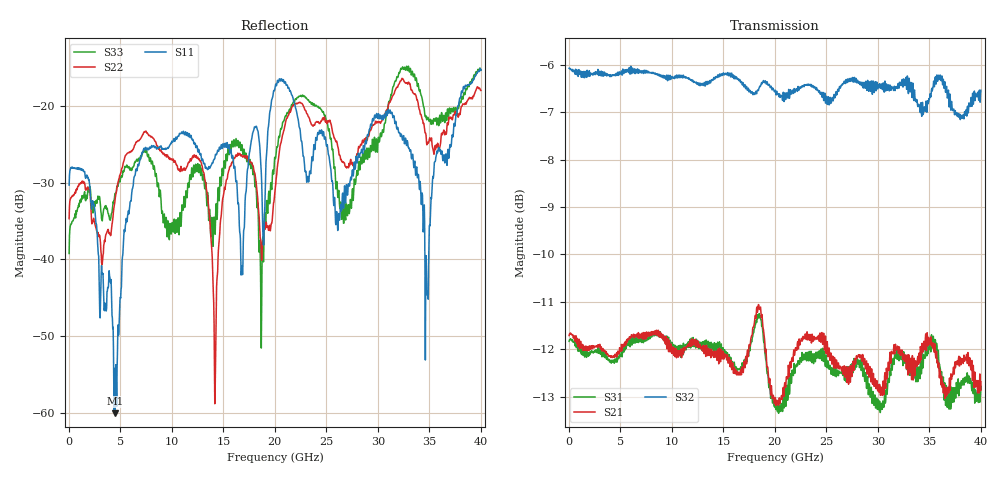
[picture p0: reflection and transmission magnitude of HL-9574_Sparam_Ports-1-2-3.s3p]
# GHZ S RI R 50.0
!; PortSelection: Port_123
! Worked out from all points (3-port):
!   1143 points, 35 MHz to 40.01 GHz, reference 50 ohm
!   strongest paths, dB at 35 MHz, 10.01 GHz, 20.02 GHz, 30.03 GHz, 40.01 GHz:
!     S32: -6.1, -6.2, -6.6, -6.4, -6.5
!     S21: -11.7, -12.1, -13.0, -12.7, -12.7
!     S31: -11.8, -11.9, -13.1, -13.1, -12.8
!   lowest |S11| = -60.1 dB at 4.48 GHz (marker M1), VSWR 1.00, Z = 50.1 - j0.0158 ohm
!   |S11| at or under -10 dB: start of sweep to end of sweep
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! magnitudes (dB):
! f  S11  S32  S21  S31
! 35 MHz  -30.3  -6.1  -11.7  -11.8
! 4.48 GHz  -60.1  -6.2  -12.1  -12.2
! 7.245 GHz  -25.7  -6.2  -11.6  -11.9
! 12.81 GHz  -26.2  -6.4  -12.0  -12.0
! 14.18 GHz  -26.9  -6.3  -12.1  -12.0
! 16.8 GHz  -40.8  -6.4  -12.5  -12.4
! 20.02 GHz  -17.6  -6.6  -13.0  -13.1
! 31.32 GHz  -20.9  -6.5  -12.0  -12.2
! 34.76 GHz  -44.4  -7.0  -11.8  -12.1
! 40.01 GHz  -15.4  -6.5  -12.7  -12.8
